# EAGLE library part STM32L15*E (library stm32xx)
STM32L1_Med_density_LQFP100 edit this description Auto generated by make-symbol-device-package-bsdl.ulp Rev. 44 Source: STM32L1_Med_density_LQFP100.bsd
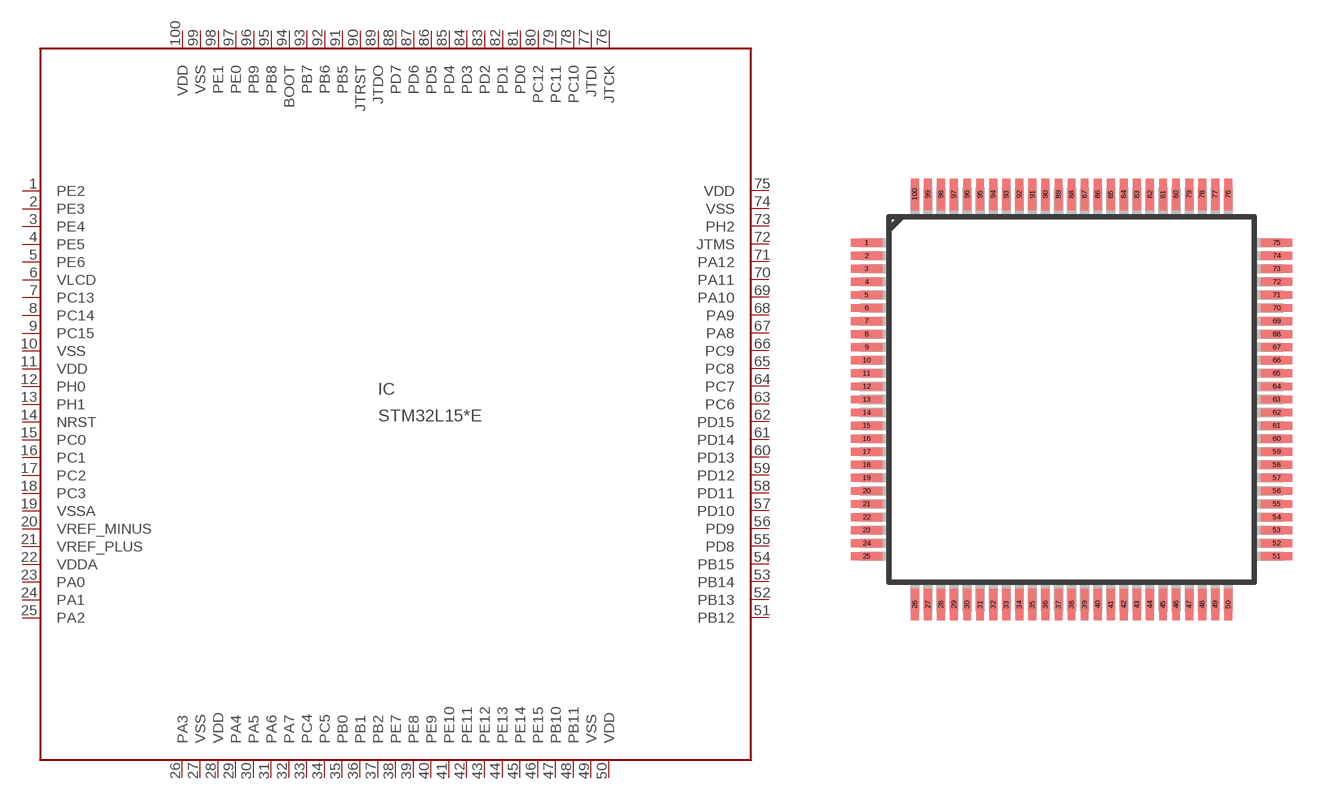
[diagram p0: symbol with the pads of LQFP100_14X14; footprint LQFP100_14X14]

Designator prefix IC

## STM32L151QE, STM32L151RE, STM32L151VE, STM32L151ZE, STM32L152QE, STM32L152RE, STM32L152VE, STM32L152ZE  [LQFP100_14X14]
1  PE2
2  PE3
3  PE4
4  PE5
5  PE6
6  VLCD  pas
7  PC13
8  PC14
9  PC15
10  VSS  pwr
11  VDD  pwr
12  PH0
13  PH1
14  NRST  in
15  PC0
16  PC1
17  PC2
18  PC3
19  VSSA  pwr
20  VREF_MINUS  pas
21  VREF_PLUS  pas
22  VDDA  pwr
23  PA0
24  PA1
25  PA2
26  PA3
27  VSS  pwr
28  VDD  pwr
29  PA4
30  PA5
31  PA6
32  PA7
33  PC4
34  PC5
35  PB0
36  PB1
37  PB2
38  PE7
39  PE8
40  PE9
41  PE10
42  PE11
43  PE12
44  PE13
45  PE14
46  PE15
47  PB10
48  PB11
49  VSS  pwr
50  VDD  pwr
51  PB12
52  PB13
53  PB14
54  PB15
55  PD8
56  PD9
57  PD10
58  PD11
59  PD12
60  PD13
61  PD14
62  PD15
63  PC6
64  PC7
65  PC8
66  PC9
67  PA8
68  PA9
69  PA10
70  PA11
71  PA12
72  JTMS  in
73  PH2
74  VSS  pwr
75  VDD  pwr
76  JTCK  in
77  JTDI  in
78  PC10
79  PC11
80  PC12
81  PD0
82  PD1
83  PD2
84  PD3
85  PD4
86  PD5
87  PD6
88  PD7
89  JTDO  out
90  JTRST  in
91  PB5
92  PB6
93  PB7
94  BOOT  in
95  PB8
96  PB9
97  PE0
98  PE1
99  VSS  pwr
100  VDD  pwr

## Footprint LQFP100_14X14 (pad centres in mm)
LQFP100_PACKAGE Auto generated by make-symbol-device-package-bsdl.ulp Rev. 44
smd 1.2 x 0.3: 1 -7.85,6; 2 -7.85,5.5; 3 -7.85,5; 4 -7.85,4.5; 5 -7.85,4; 6 -7.85,3.5; 7 -7.85,3; 8 -7.85,2.5; 9 -7.85,2; 10 -7.85,1.5; 11 -7.85,1; 12 -7.85,0.5; 13 -7.85,0; 14 -7.85,-0.5; 15 -7.85,-1; 16 -7.85,-1.5; 17 -7.85,-2; 18 -7.85,-2.5; 19 -7.85,-3; 20 -7.85,-3.5; 21 -7.85,-4; 22 -7.85,-4.5; 23 -7.85,-5; 24 -7.85,-5.5; 25 -7.85,-6; 51 7.85,-6; 52 7.85,-5.5; 53 7.85,-5; 54 7.85,-4.5; 55 7.85,-4; 56 7.85,-3.5; 57 7.85,-3; 58 7.85,-2.5; 59 7.85,-2; 60 7.85,-1.5; 61 7.85,-1; 62 7.85,-0.5; 63 7.85,0; 64 7.85,0.5; 65 7.85,1; 66 7.85,1.5; 67 7.85,2; 68 7.85,2.5; 69 7.85,3; 70 7.85,3.5; 71 7.85,4; 72 7.85,4.5; 73 7.85,5; 74 7.85,5.5; 75 7.85,6
smd 0.3 x 1.2: 26 -6,-7.85; 27 -5.5,-7.85; 28 -5,-7.85; 29 -4.5,-7.85; 30 -4,-7.85; 31 -3.5,-7.85; 32 -3,-7.85; 33 -2.5,-7.85; 34 -2,-7.85; 35 -1.5,-7.85; 36 -1,-7.85; 37 -0.5,-7.85; 38 0,-7.85; 39 0.5,-7.85; 40 1,-7.85; 41 1.5,-7.85; 42 2,-7.85; 43 2.5,-7.85; 44 3,-7.85; 45 3.5,-7.85; 46 4,-7.85; 47 4.5,-7.85; 48 5,-7.85; 49 5.5,-7.85; 50 6,-7.85; 76 6,7.85; 77 5.5,7.85; 78 5,7.85; 79 4.5,7.85; 80 4,7.85; 81 3.5,7.85; 82 3,7.85; 83 2.5,7.85; 84 2,7.85; 85 1.5,7.85; 86 1,7.85; 87 0.5,7.85; 88 0,7.85; 89 -0.5,7.85; 90 -1,7.85; 91 -1.5,7.85; 92 -2,7.85; 93 -2.5,7.85; 94 -3,7.85; 95 -3.5,7.85; 96 -4,7.85; 97 -4.5,7.85; 98 -5,7.85; 99 -5.5,7.85; 100 -6,7.85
